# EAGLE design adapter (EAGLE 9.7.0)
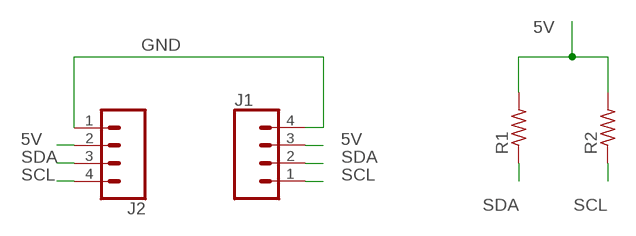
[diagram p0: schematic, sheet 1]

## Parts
J1  CONN_04LONGPADS  [1X04_LONGPADS]
J2  CONN_04LONGPADS  [1X04_LONGPADS]
R1  RES-US1206FAB  [R1206FAB]
R2  RES-US1206FAB  [R1206FAB]

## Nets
5V: J1.3 J2.2 R1.2 R2.2
GND: J1.4 J2.1
SCL: J1.1 J2.4 R2.1
SDA: J1.2 J2.3 R1.1

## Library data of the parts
J1 J2 = SparkFun-Connectors:CONN_04: Multi connection point. Often used as Generic Header-pin footprint for 0.1 inch spaced/style header connections On any of the 0.1 inch spaced packages, you can populate with these: Break Away Headers - Straight (PRT-00116) Break Away Male Headers - Right Angle (PRT-00553) Female Headers (PRT-00115)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; PROD_ID: CONN-09696
R1 R2 = fab2:RES-US: Resistor (US Symbol)

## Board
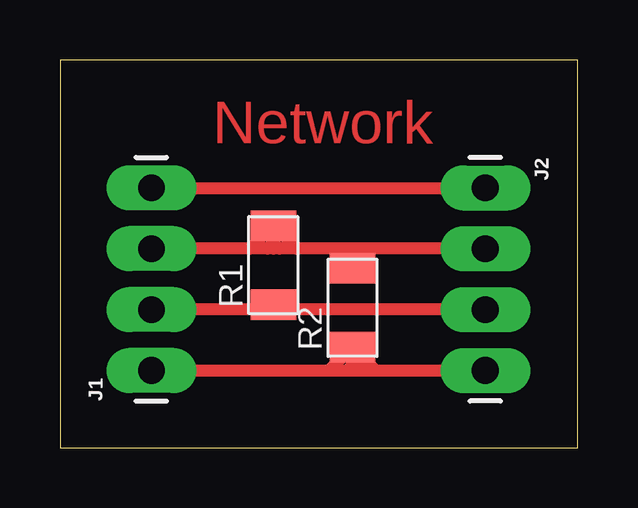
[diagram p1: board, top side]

Size 21.57 x 16.18 mm. Coordinates in mm from the lower left corner, seen from the top.
Outline: 0,0 21.57,0 21.57,16.18 0,16.18 0,0
Copper layers (1*16): Top / Bottom
Stack-up Default Layer Stack: Top User Defined 0.035mm / Dielectric-1 User Defined 1.5mm / Bottom User Defined 0.035mm
Design rules "default *": minimum track width 20mil, minimum drill 0.35mm, track to track 20mil, track to pad 6mil, pad to pad 6mil, via to via 6mil, smd to smd 6mil, copper to edge 40mil, drill to drill 6mil, minimum pad ring 10mil, minimum via ring 8mil, stop-mask expansion 4mil, vias tented up to drill 0mil, thermal gap 10mil

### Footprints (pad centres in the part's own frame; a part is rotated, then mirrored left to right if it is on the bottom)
1X04_LONGPADS = drill 1.118 pad 1.88 long: 1 0,0; 2 2.54,0; 3 5.08,0; 4 7.62,0
R1206FAB = smd 1.27 x 1.905: 1 -1.651,0; 2 1.651,0

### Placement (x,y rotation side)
J1  3.81,3.23 90 top
J2  17.72,10.85 270 top
R1  8.89,7.62 90 top
R2  12.19,5.84 90 top

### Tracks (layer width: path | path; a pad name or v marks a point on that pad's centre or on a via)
5V
  Top 0.508: 11.94,7.49 R2.2 12.19,8.31 | J2.2 12.19,8.31 | 12.19,8.31 9.86,8.31 | 9.86,8.31 9.14,8.31 | 9.14,8.31 8.89,8.31 | 8.89,8.31 8.64,8.31 | 8.64,8.31 7.92,8.31 | 7.92,8.31 J1.3 | R1.2 8.89,8.31 | R1.2 9.86,8.31 | R1.2 7.92,8.31 | 8.89,8.56 8.64,8.31 | R1.2 8.89,8.56 | 8.89,8.56 9.14,8.31
GND
  Top 0.508: J1.4 J2.1
SCL
  Top 0.508: J1.1 11.23,3.23 | 11.23,3.23 11.94,3.23 | 11.94,3.23 12.19,3.23 | 12.19,3.23 12.45,3.23 | 12.45,3.23 13.16,3.23 | 13.16,3.23 J2.4 | R2.1 12.19,3.23 | R2.1 11.23,3.23 | R2.1 13.16,3.23 | R2.1 12.45,3.94 12.45,3.23 | R2.1 12.19,3.48 11.94,3.23
SDA
  Top 0.508: J2.3 8.89,5.77 | 8.89,5.77 J1.2 | R1.1 8.89,5.77

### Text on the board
Top: Network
